| TEXAS INSTRUMENTS INCORPORATED
| Standard Linear and Logic Group
| IBIS Model of SN74CBT16244
| 16-BIT FET BUS SWITCHES
| This file contains package information for the following:
|  TSSOP 48-pin (DGG) package as [Component] CBT16244_DGG
|  TVSOP 48-pin (DGV) package as [Component] CBT16244_DGV
|  SSOP 48-pin (DL) package as [Component] CBT16244_DL
| This device can be powered at the following Vccs:
|  4 volt Vcc
|  5 volt Vcc
| This file provides unique models under the [Model Selector] for each Vcc.
| For operation at a specific Vcc, select the appropriate model after each
| [Model Selector] keyword.
[IBIS Ver]   3.2
[Comment char]  |_char
[File Name]   sn74cbt16244.ibs
[File Rev]   1.1 | e_die
[Date]   January 17, 2003
[Source]   Data created from TI-SPICE simulations at TI-SLL.
[Notes]   The following is an IBIS list for the CBT16244.
   Please contact sllibis@ti.com with questions and
   comments concerning SLL IBIS models.
   - Power-clamp data has been deleted since there is no
   power-clamp diode in the device.
   - Non-monotonic data due to device characteristics.
[Disclaimer] Property of Texas Instruments Incorporated.  Unauthorized
   reproduction and/or distribution is strictly prohibited.
   This product is protected under copyright law.
   Created  2003, (C) Copyright  2003, Texas Instruments
   Incorporated, All Rights Reserved
   UNLESS THERE IS A SIGNED, WRITTEN AGREEMENT TO THE
   CONTRARY, TEXAS INSTRUMENTS (TI) IS PROVIDING THE IBIS
   MODELS  AND WITHOUT ANY WARRANTY, EXPRESSED OR
   IMPLIED.  TI assumes no liability for:
   1) the accuracy of the IBIS models provided to your
   company;
   2) the proper functioning of these IBIS Models in your
   design or for any resulting applications; or
   3) infringement of patents, copyrights or intellectual
   property rights resulting from your use of these IBIS
   models.
   TI provides IBIS Models as a service to our customers.
   You and your company shall not distribute, sell or give
   these models to anyone else without prior written
   permission from TI.
   TI reserves the right to make changes to our products or
   to discontinue any semiconductor product or service
   without notice, and advises our customers to obtain the
   latest version of relevant information to verify, before
   placing orders, that the information being relied on is
   current.
   Please be aware that your receipt and use of the IBIS
   information provided shall serve as acceptance of these
   terms and conditions.  If you do not accept these terms,
   you should return or destroy the IBIS models and any
   other accompanying information immediately.
| Component CBT16244_DGG 48-pin TSSOP
[Component]   CBT16244_DGG
[Manufacturer]   Texas Instruments, Inc.
[Package]
|   typ   min   max
R_pkg   4.400e-02   3.800e-02   5.100e-02
L_pkg   3.019e-09   2.486e-09   4.099e-09
C_pkg   5.070e-13   3.340e-13   8.090e-13
[Pin]   signal_name   model_name   R_pin   L_pin   C_pin
1   1NOE   CBT16244_NOE   4.100e-02   4.017e-09   7.590e-13
2   1B1   CBT16244_IO   4.200e-02   3.737e-09   7.920e-13
3   1B2   CBT16244_IO   4.200e-02   3.480e-09   6.610e-13
4   GND   GND   3.800e-02   3.131e-09   5.750e-13
5   1B3   CBT16244_IO   4.700e-02   3.122e-09   5.660e-13
6   1B4   CBT16244_IO   4.300e-02   2.948e-09   5.040e-13
7   VCC   POWER   4.500e-02   2.845e-09   3.970e-13
8   2B1   CBT16244_IO   4.900e-02   2.835e-09   3.940e-13
9   2B2   CBT16244_IO   4.800e-02   2.715e-09   3.780e-13
10   GND   GND   5.000e-02   2.664e-09   3.630e-13
11   2B3   CBT16244_IO   5.000e-02   2.585e-09   3.480e-13
12   2B4   CBT16244_IO   4.900e-02   2.550e-09   3.370e-13
13   3B1   CBT16244_IO   4.900e-02   2.541e-09   3.360e-13
14   3B2   CBT16244_IO   5.000e-02   2.574e-09   3.480e-13
15   GND   GND   4.900e-02   2.618e-09   3.590e-13
16   3B3   CBT16244_IO   4.600e-02   2.671e-09   3.750e-13
17   3B4   CBT16244_IO   4.500e-02   2.754e-09   3.890e-13
18   VCC   POWER   4.400e-02   2.823e-09   4.500e-13
19   4B1   CBT16244_IO   4.200e-02   2.968e-09   5.030e-13
20   4B2   CBT16244_IO   5.100e-02   3.108e-09   5.350e-13
21   GND   GND   4.200e-02   3.175e-09   5.870e-13
22   4B3   CBT16244_IO   4.100e-02   3.449e-09   6.780e-13
23   4B4   CBT16244_IO   4.400e-02   3.766e-09   8.040e-13
24   4NOE   CBT16244_NOE   4.300e-02   4.065e-09   7.610e-13
25   3NOE   CBT16244_NOE   4.100e-02   3.994e-09   7.570e-13
26   4A4   CBT16244_IO   3.900e-02   3.649e-09   7.890e-13
27   4A3   CBT16244_IO   3.800e-02   3.362e-09   6.600e-13
28   GND   GND   3.800e-02   3.082e-09   5.740e-13
29   4A2   CBT16244_IO   4.400e-02   2.990e-09   5.220e-13
30   4A1   CBT16244_IO   4.100e-02   2.917e-09   4.950e-13
31   VCC   POWER   4.300e-02   2.820e-09   4.480e-13
32   3A4   CBT16244_IO   4.300e-02   2.699e-09   3.850e-13
33   3A3   CBT16244_IO   4.500e-02   2.628e-09   3.720e-13
34   GND   GND   4.600e-02   2.556e-09   3.560e-13
35   3A2   CBT16244_IO   4.600e-02   2.495e-09   3.440e-13
36   3A1   CBT16244_IO   4.700e-02   2.487e-09   3.340e-13
37   2A4   CBT16244_IO   4.700e-02   2.490e-09   3.350e-13
38   2A3   CBT16244_IO   4.600e-02   2.486e-09   3.430e-13
39   GND   GND   4.500e-02   2.566e-09   3.560e-13
40   2A2   CBT16244_IO   4.400e-02   2.639e-09   3.740e-13
41   2A1   CBT16244_IO   4.300e-02   2.701e-09   3.860e-13
42   VCC   POWER   4.300e-02   2.817e-09   4.500e-13
43   1A4   CBT16244_IO   4.100e-02   2.935e-09   5.010e-13
44   1A3   CBT16244_IO   4.700e-02   3.035e-09   5.290e-13
45   GND   GND   4.300e-02   3.171e-09   5.890e-13
46   1A2   CBT16244_IO   4.000e-02   3.415e-09   6.820e-13
47   1A1   CBT16244_IO   4.300e-02   3.741e-09   8.090e-13
48   2NOE   CBT16244_NOE   4.400e-02   4.099e-09   7.640e-13
| Component CBT16244_DGV 48-pin TVSOP
[Component]   CBT16244_DGV
[Manufacturer]   Texas Instruments, Inc.
[Package]
|   typ   min   max
R_pkg   7.000e-02   4.900e-02   8.500e-02
L_pkg   3.013e-09   2.743e-09   3.408e-09
C_pkg   3.710e-13   2.940e-13   5.110e-13
[Pin]   signal_name   model_name   R_pin   L_pin   C_pin
1   1NOE   CBT16244_NOE   4.900e-02   3.393e-09   4.970e-13
2   1B1   CBT16244_IO   6.000e-02   3.250e-09   5.020e-13
3   1B2   CBT16244_IO   7.700e-02   3.310e-09   4.510e-13
4   GND   GND   8.500e-02   3.299e-09   4.040e-13
5   1B3   CBT16244_IO   8.300e-02   3.136e-09   3.600e-13
6   1B4   CBT16244_IO   7.700e-02   3.019e-09   3.630e-13
7   VCC   POWER   6.500e-02   2.882e-09   3.490e-13
8   2B1   CBT16244_IO   6.600e-02   2.829e-09   3.140e-13
9   2B2   CBT16244_IO   6.700e-02   2.796e-09   3.140e-13
10   GND   GND   6.900e-02   2.754e-09   3.080e-13
11   2B3   CBT16244_IO   7.000e-02   2.753e-09   3.010e-13
12   2B4   CBT16244_IO   7.100e-02   2.745e-09   2.940e-13
13   3B1   CBT16244_IO   7.000e-02   2.744e-09   2.940e-13
14   3B2   CBT16244_IO   7.000e-02   2.754e-09   3.010e-13
15   GND   GND   6.900e-02   2.754e-09   3.080e-13
16   3B3   CBT16244_IO   6.700e-02   2.796e-09   3.140e-13
17   3B4   CBT16244_IO   6.600e-02   2.829e-09   3.140e-13
18   VCC   POWER   6.500e-02   2.883e-09   3.500e-13
19   4B1   CBT16244_IO   7.500e-02   3.014e-09   3.630e-13
20   4B2   CBT16244_IO   8.000e-02   3.128e-09   3.580e-13
21   GND   GND   8.400e-02   3.295e-09   4.030e-13
22   4B3   CBT16244_IO   7.800e-02   3.311e-09   4.520e-13
23   4B4   CBT16244_IO   6.200e-02   3.259e-09   5.010e-13
24   4NOE   CBT16244_NOE   5.200e-02   3.404e-09   4.960e-13
25   3NOE   CBT16244_NOE   5.300e-02   3.397e-09   5.050e-13
26   4A4   CBT16244_IO   6.200e-02   3.249e-09   5.110e-13
27   4A3   CBT16244_IO   7.700e-02   3.308e-09   4.530e-13
28   GND   GND   8.200e-02   3.289e-09   4.030e-13
29   4A2   CBT16244_IO   7.800e-02   3.121e-09   3.590e-13
30   4A1   CBT16244_IO   7.400e-02   3.010e-09   3.630e-13
31   VCC   POWER   6.500e-02   2.883e-09   3.490e-13
32   3A4   CBT16244_IO   6.700e-02   2.829e-09   3.140e-13
33   3A3   CBT16244_IO   6.700e-02   2.795e-09   3.140e-13
34   GND   GND   6.900e-02   2.753e-09   3.070e-13
35   3A2   CBT16244_IO   7.000e-02   2.753e-09   3.010e-13
36   3A1   CBT16244_IO   7.000e-02   2.743e-09   2.940e-13
37   2A4   CBT16244_IO   7.000e-02   2.743e-09   2.940e-13
38   2A3   CBT16244_IO   7.000e-02   2.753e-09   3.010e-13
39   GND   GND   6.900e-02   2.754e-09   3.070e-13
40   2A2   CBT16244_IO   6.800e-02   2.797e-09   3.140e-13
41   2A1   CBT16244_IO   6.700e-02   2.830e-09   3.140e-13
42   VCC   POWER   6.400e-02   2.880e-09   3.490e-13
43   1A4   CBT16244_IO   7.200e-02   3.004e-09   3.620e-13
44   1A3   CBT16244_IO   7.800e-02   3.121e-09   3.590e-13
45   GND   GND   8.400e-02   3.296e-09   4.030e-13
46   1A2   CBT16244_IO   7.700e-02   3.308e-09   4.510e-13
47   1A1   CBT16244_IO   6.200e-02   3.258e-09   4.990e-13
48   2NOE   CBT16244_NOE   5.300e-02   3.408e-09   4.940e-13
| Component CBT16244 48-pin SSOP
[Component]   CBT16244
[Manufacturer]   Texas Instruments, Inc.
[Package]
|   typ   min   max
R_pkg   4.800e-02   3.800e-02   5.300e-02
L_pkg   6.046e-09   5.084e-09   7.968e-09
C_pkg   8.130e-13   5.690e-13   1.157e-12
[Pin]   signal_name   model_name   R_pin   L_pin   C_pin
1   1NOE   CBT16244_NOE   4.600e-02   7.968e-09   1.017e-12
2   1B1   CBT16244_IO   4.400e-02   7.299e-09   1.157e-12
3   1B2   CBT16244_IO   4.300e-02   6.765e-09   1.058e-12
4   GND   GND   4.100e-02   6.269e-09   9.330e-13
5   1B3   CBT16244_IO   3.800e-02   5.856e-09   8.290e-13
6   1B4   CBT16244_IO   4.600e-02   5.802e-09   7.900e-13
7   VCC   POWER   5.000e-02   5.656e-09   7.380e-13
8   2B1   CBT16244_IO   5.300e-02   5.500e-09   6.430e-13
9   2B2   CBT16244_IO   5.200e-02   5.304e-09   6.060e-13
10   GND   GND   5.300e-02   5.189e-09   5.830e-13
11   2B3   CBT16244_IO   5.100e-02   5.084e-09   5.690e-13
12   2B4   CBT16244_IO   5.300e-02   5.862e-09   8.330e-13
13   3B1   CBT16244_IO   5.300e-02   5.862e-09   8.330e-13
14   3B2   CBT16244_IO   5.100e-02   5.084e-09   5.690e-13
15   GND   GND   5.300e-02   5.189e-09   5.830e-13
16   3B3   CBT16244_IO   5.200e-02   5.304e-09   6.060e-13
17   3B4   CBT16244_IO   5.300e-02   5.500e-09   6.430e-13
18   VCC   POWER   5.000e-02   5.656e-09   7.380e-13
19   4B1   CBT16244_IO   4.600e-02   5.802e-09   7.900e-13
20   4B2   CBT16244_IO   3.800e-02   5.856e-09   8.290e-13
21   GND   GND   4.100e-02   6.269e-09   9.330e-13
22   4B3   CBT16244_IO   4.300e-02   6.765e-09   1.058e-12
23   4B4   CBT16244_IO   4.400e-02   7.299e-09   1.157e-12
24   4NOE   CBT16244_NOE   4.600e-02   7.968e-09   1.017e-12
25   3NOE   CBT16244_NOE   4.600e-02   7.968e-09   1.017e-12
26   4A4   CBT16244_IO   4.400e-02   7.299e-09   1.157e-12
27   4A3   CBT16244_IO   4.300e-02   6.765e-09   1.058e-12
28   GND   GND   4.100e-02   6.269e-09   9.330e-13
29   4A2   CBT16244_IO   3.800e-02   5.856e-09   8.290e-13
30   4A1   CBT16244_IO   4.600e-02   5.802e-09   7.900e-13
31   VCC   POWER   5.000e-02   5.656e-09   7.380e-13
32   3A4   CBT16244_IO   5.300e-02   5.500e-09   6.430e-13
33   3A3   CBT16244_IO   5.200e-02   5.304e-09   6.060e-13
34   GND   GND   5.300e-02   5.189e-09   5.830e-13
35   3A2   CBT16244_IO   5.100e-02   5.084e-09   5.690e-13
36   3A1   CBT16244_IO   5.300e-02   5.862e-09   8.330e-13
37   2A4   CBT16244_IO   5.300e-02   5.862e-09   8.330e-13
38   2A3   CBT16244_IO   5.100e-02   5.084e-09   5.690e-13
39   GND   GND   5.300e-02   5.189e-09   5.830e-13
40   2A2   CBT16244_IO   5.200e-02   5.304e-09   6.060e-13
41   2A1   CBT16244_IO   5.300e-02   5.500e-09   6.430e-13
42   VCC   POWER   5.000e-02   5.656e-09   7.380e-13
43   1A4   CBT16244_IO   4.600e-02   5.802e-09   7.900e-13
44   1A3   CBT16244_IO   3.800e-02   5.856e-09   8.290e-13
45   GND   GND   4.100e-02   6.269e-09   9.330e-13
46   1A2   CBT16244_IO   4.300e-02   6.765e-09   1.058e-12
47   1A1   CBT16244_IO   4.400e-02   7.299e-09   1.157e-12
48   2NOE   CBT16244_NOE   4.600e-02   7.967e-09   1.017e-12
[Series Switch Groups]
| Function Group States
On  1 /   | 1A1-1A4->1B1-1B4 1NOE LOW
On  2 /   | 2A1-2A4->2B1-2B4 2NOE LOW
On  3 /   | 3A1-3A4->3B1-3B4 3NOE LOW
On  4 /   | 4A1-4A4->4B1-4B4 4NOE LOW
On  1 2 /   | Enable Both
On  1 3 /   | Enable Both
On  1 4 /   | Enable Both
On  2 3 /   | Enable Both
On  2 4 /   | Enable Both
On  3 4 /   | Enable Both
On  1 2 3 /   | Enable 1 2 3
On  1 2 4 /   | Enable 1 2 4
On  1 3 4 /   | Enable 1 3 4
On  2 3 4 /   | Enable 2 3 4
On  1 2 3 4 /   | Enable All
[Series Pin Mapping]   pin_2   model_name   function_table_group
43   6   CBT16244_IO_40_S   1
| 43   6   CBT16244_IO_50_S   1
44   5   CBT16244_IO_40_S   1
| 44   5   CBT16244_IO_50_S   1
46   3   CBT16244_IO_40_S   1
| 46   3   CBT16244_IO_50_S   1
47   2   CBT16244_IO_40_S   1
| 47   2   CBT16244_IO_50_S   1
37   12   CBT16244_IO_40_S   2
| 37   12   CBT16244_IO_50_S   2
38   11   CBT16244_IO_40_S   2
| 38   11   CBT16244_IO_50_S   2
40   9   CBT16244_IO_40_S   2
| 40   9   CBT16244_IO_50_S   2
41   8   CBT16244_IO_40_S   2
| 41   8   CBT16244_IO_50_S   2
32   17   CBT16244_IO_40_S   3
| 32   17   CBT16244_IO_50_S   3
33   16   CBT16244_IO_40_S   3
| 33   16   CBT16244_IO_50_S   3
35   14   CBT16244_IO_40_S   3
| 35   14   CBT16244_IO_50_S   3
36   13   CBT16244_IO_40_S   3
| 36   13   CBT16244_IO_50_S   3
26   23   CBT16244_IO_40_S   4
| 26   23   CBT16244_IO_50_S   4
27   22   CBT16244_IO_40_S   4
| 27   22   CBT16244_IO_50_S   4
29   20   CBT16244_IO_40_S   4
| 29   20   CBT16244_IO_50_S   4
30   19   CBT16244_IO_40_S   4
| 30   19   CBT16244_IO_50_S   4
| Model CBT16244_NOE
[Model Selector]   CBT16244_NOE
CBT16244_NOE_40   4 volt Vcc
CBT16244_NOE_50   5 volt Vcc
| Model CBT16244_IO
[Model Selector]   CBT16244_IO
CBT16244_IO_40   4 volt Vcc
CBT16244_IO_50   5 volt Vcc
| Model CBT16244_IO_S
[Model Selector]   CBT16244_IO_S
CBT16244_IO_40_S   4 volt Vcc
CBT16244_IO_50_S   5 volt Vcc
[Model]   CBT16244_IO_40_S
Model_type  Series_switch
| variable   typ   min   max
C_comp   0   0   0
[Temperature Range]   40   100   -40
| Ambient temperature   25   85   -40
[Voltage range]   4   4   4
[On]
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[Off]
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[Model]   CBT16244_IO_50_S
Model_type  Series_switch
| variable   typ   min   max
C_comp   0   0   0
[Temperature Range]   40   100   -40
| Ambient temperature   25   85   -40
[Voltage range]   5   4.5   5.5
[On]
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[Off]
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| Models and submodels in the file (6): CBT16244_NOE_40 (Input), CBT16244_NOE_50 (Input), CBT16244_IO_40_S (Series_switch), CBT16244_IO_40 (Terminator), CBT16244_IO_50_S (Series_switch), CBT16244_IO_50 (Terminator)
